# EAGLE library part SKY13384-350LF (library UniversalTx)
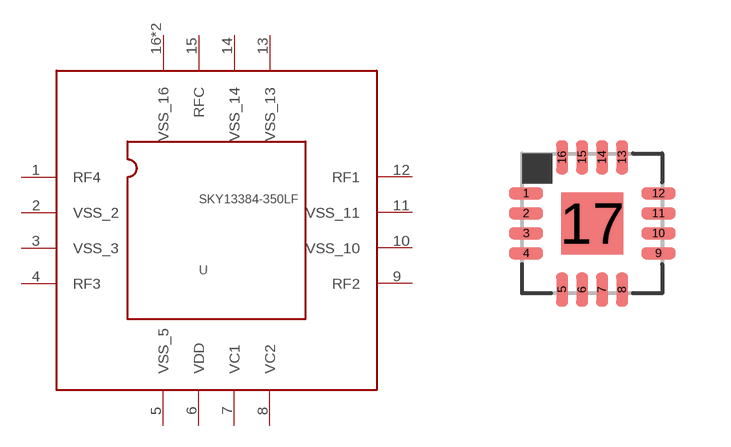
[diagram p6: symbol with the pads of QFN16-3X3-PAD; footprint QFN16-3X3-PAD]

Designator prefix -

## SKY13384-350LF  [QFN16-3X3-PAD]
1  RF4
2  VSS_2
3  VSS_3
4  RF3
5  VSS_5
6  VDD
7  VC1
8  VC2
9  RF2
10  VSS_10
11  VSS_11
12  RF1
13  VSS_13
14  VSS_14
15  RFC
16  VSS_16
17  VSS_16

## Footprint QFN16-3X3-PAD (pad centres in mm)
RTE (S-PQFP-N16) 3x3 mm Source: www.ti.com .. tpa6132a2 direct path stereo $.65.pdf
smd 0.85 x 0.3: 1 -1.655,0.75; 2 -1.655,0.25; 3 -1.655,-0.25; 4 -1.655,-0.75; 9 1.655,-0.75; 10 1.655,-0.25; 11 1.655,0.25; 12 1.655,0.75
smd 0.3 x 0.85: 5 -0.75,-1.655; 6 -0.25,-1.655; 7 0.25,-1.655; 8 0.75,-1.655; 13 0.75,1.655; 14 0.25,1.655; 15 -0.25,1.655; 16 -0.75,1.655
smd 1.55 x 1.55: 17 0,0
